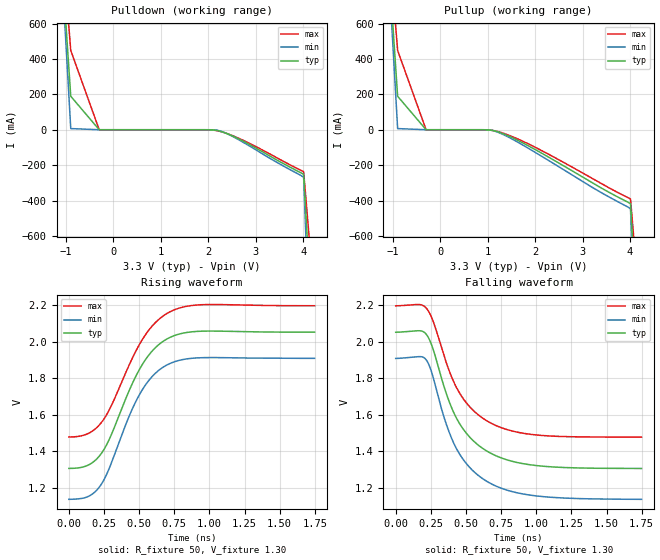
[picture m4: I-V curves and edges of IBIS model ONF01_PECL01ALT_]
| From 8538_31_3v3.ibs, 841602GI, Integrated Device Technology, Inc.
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[Model]   ONF01_PECL01ALT_
Model_type   Output_ECL
Polarity   Non-Inverting
|   typ   min   max
C_comp   2pF   1.5pF   2.5pF
Vmeas = 1.65V
Rref = 50
Cref = 0
Vref = 1.3V
|   typ   min   max
[Voltage range]   3.3V   3.135V   3.465V
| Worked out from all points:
|   rising waveform, R_fixture 50, V_fixture 1.30: 20-80 % time 265ps typ, 258ps min, 275ps max; typ from 1.3 V to 2.05 V
|   falling waveform, R_fixture 50, V_fixture 1.30: 20-80 % time 267ps typ, 268ps min, 262ps max; typ from 2.05 V to 1.31 V
[Pulldown]
|Voltage   I (typ)   I (min)   I (max)
-3.3V     9.786A     12.03A     8.45A
-1.5V     2.58A      2.839A     2.441A
-900mV    189.2mA    6.554mA    448mA
-300mV    38.6nA     139.1pA    1.11uA
1.978V    -72.1uA    -11.25uA   -210.2uA
2.176V    -3.776mA   -2.26mA    -4.928mA
2.274V    -10.4mA    -9.107mA   -11.2mA
2.471V    -30.54mA   -32.27mA   -29.14mA
2.817V    -76.23mA   -83.67mA   -70.15mA
4.01V     -251.5mA   -269.3mA   -237mA
4.528V    -2.679A    -3.924A    -1.886A
6.6V      -15.69A    -20.55A    -12.73A
[Pullup]
|Voltage   I (typ)   I (min)   I (max)
-3.3V     9.786A     12.03A     8.45A
-1.5V     2.58A      2.839A     2.441A
-900mV    189.2mA    6.554mA    448mA
-300mV    38.6nA     139.1pA    1.11uA
1.041V    -1.703mA   -1.46mA    -1.795mA
1.288V    -18.86mA   -22.48mA   -16.27mA
1.682V    -66.67mA   -77.83mA   -57.93mA
2.274V    -153.5mA   -172.3mA   -137.3mA
3.26V     -308.3mA   -334.7mA   -283.7mA
4.01V     -417.3mA   -447.3mA   -391.2mA
4.528V    -2.844A    -4.101A    -2.041A
6.6V      -15.79A    -20.6A     -12.84A
[Ramp]
|   typ   min   max
dV/dt_r   0.602/0.413n   0.621/0.4n   0.58/0.429n
dV/dt_f   0.603/0.442n   0.625/0.444n   0.581/0.431n
R_load =   50.0000
[Rising Waveform]
R_fixture = 50
V_fixture = 1.30   | VCC_typ - 2V
V_fixture_max = 1.465   | VCC_max - 2V
V_fixture_min = 1.135   | VCC_min - 2V
C_fixture = 0.0p
| Time   typ   min   max
0s        1.305V     1.136V     1.478V
133.1ps   1.322V     1.15V      1.495V
220.7ps   1.376V     1.207V     1.547V
296ps     1.479V     1.322V     1.639V
416.9ps   1.71V      1.569V     1.851V
495.7ps   1.839V     1.7V       1.976V
583.3ps   1.94V      1.801V     2.077V
684.9ps   2.009V     1.867V     2.148V
933.7ps   2.057V     1.912V     2.202V
1.748ns   2.052V     1.909V     2.197V
[Falling Waveform]
R_fixture = 50
V_fixture = 1.30   | VCC_typ - 2V
V_fixture_max = 1.465   | VCC_max - 2V
V_fixture_min = 1.135   | VCC_min - 2V
C_fixture = 0.0p
| Time   typ   min   max
0s        2.052V     1.909V     2.197V
171.7ps   2.06V      1.919V     2.204V
217.2ps   2.041V     1.901V     2.185V
266.3ps   1.959V     1.806V     2.113V
348.6ps   1.743V     1.575V     1.912V
423.9ps   1.594V     1.427V     1.762V
525.5ps   1.478V     1.312V     1.645V
656.9ps   1.397V     1.231V     1.563V
993.2ps   1.322V     1.156V     1.49V
1.748ns   1.306V     1.137V     1.478V
